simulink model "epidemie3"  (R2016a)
settings: Solver=FixedStepDiscrete  StartTime=0.0  StopTime=300  FixedStep=1  RelTol=1e-3
InitFcn:
  | init_epidemie
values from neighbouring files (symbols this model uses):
  dt = block.DialogPrm(4).Data    [sfun_oven.m]
  m = 1.0    (= 1)    [init_pendelStange.m]
undefined symbols (not defined in the file or in its folder): N0, v

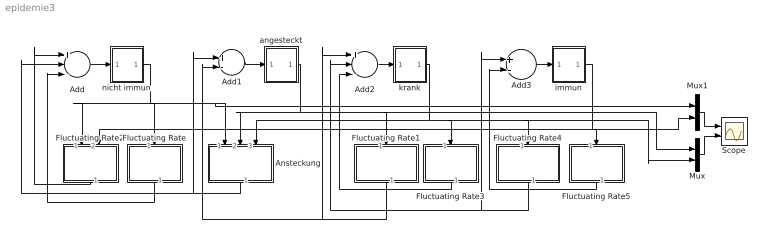
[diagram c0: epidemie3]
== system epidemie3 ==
  Add : Sum  Inputs=+--
  Add1 : Sum  Inputs=+-
  Add2 : Sum  Inputs=+--
  Add3 : Sum  Inputs=+-
  Ansteckung : Subsystem
  Fluctuating Rate : Subsystem
  Fluctuating Rate1 : Subsystem
  Fluctuating Rate2 : Subsystem
  Fluctuating Rate3 : Subsystem
  Fluctuating Rate4 : Subsystem
  Fluctuating Rate5 : Subsystem
  Mux : Mux  Inputs=2
  Mux1 : Mux  Inputs=2
  Scope : Scope  NumInputPorts=2
  angesteckt : Subsystem
  immun : Subsystem
  krank : Subsystem
  nicht immun : Subsystem
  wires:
  Add/1 -> nicht immun/1(In)
  nicht immun/1(Out) -> Ansteckung/1(N), Mux1/1, Fluctuating Rate/1(N), Fluctuating Rate2/1(N)
  immun/1(Out) -> Mux1/2, Fluctuating Rate5/1(N), Fluctuating Rate2/2(I)
  Fluctuating Rate2/1(dn) -> Add/1
  angesteckt/1(Out) -> Ansteckung/2(A), Mux/1, Fluctuating Rate1/1(N)
  krank/1(Out) -> Ansteckung/3(K), Mux/2, Fluctuating Rate4/1(N), Fluctuating Rate3/1(N)
  Ansteckung/1(a) -> Add/2, Add1/1
  Add1/1 -> angesteckt/1(In)
  Fluctuating Rate1/1(dn) -> Add2/1, Add1/2
  Add2/1 -> krank/1(In)
  Fluctuating Rate4/1(dn) -> Add3/1, Add2/2
  Fluctuating Rate3/1(dn) -> Add2/3
  Mux1/1 -> Scope/1
  Mux/1 -> Scope/2
  Add3/1 -> immun/1(In)
  Fluctuating Rate/1(dn) -> Add/3
  Fluctuating Rate5/1(dn) -> Add3/2

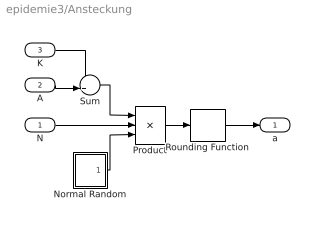
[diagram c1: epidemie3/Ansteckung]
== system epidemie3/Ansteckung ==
  N : Inport
  A : Inport  Port=2
  K : Inport  Port=3
  Normal Random : Subsystem
  Product : Product  Inputs=3
  Rounding Function : Rounding  Operator=round
  Sum : Sum  Inputs=++|
  a : Outport
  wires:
  Sum/1 -> Product/1
  Product/1 -> Rounding Function/1
  K/1 -> Sum/1
  A/1 -> Sum/2
  N/1 -> Product/2
  Normal Random/1(Out1) -> Product/3
  Rounding Function/1 -> a/1

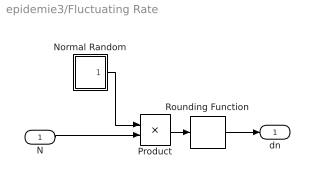
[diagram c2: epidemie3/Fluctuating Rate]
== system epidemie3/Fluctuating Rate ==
  N : Inport
  Normal Random : Subsystem
  Product : Product
  Rounding Function : Rounding  Operator=round
  dn : Outport
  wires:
  Product/1 -> Rounding Function/1
  Normal Random/1(Out1) -> Product/1
  N/1 -> Product/2
  Rounding Function/1 -> dn/1

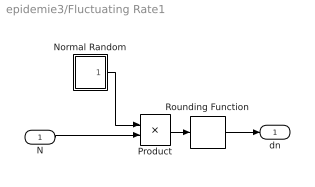
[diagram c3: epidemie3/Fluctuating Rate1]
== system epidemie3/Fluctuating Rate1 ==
  N : Inport
  Normal Random : Subsystem
  Product : Product
  Rounding Function : Rounding  Operator=round
  dn : Outport
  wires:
  Rounding Function/1 -> dn/1
  N/1 -> Product/2
  Normal Random/1(Out1) -> Product/1
  Product/1 -> Rounding Function/1

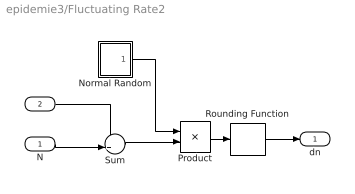
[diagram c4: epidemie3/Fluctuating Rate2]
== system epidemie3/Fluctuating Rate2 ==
  N : Inport
  I : Inport  Port=2
  Normal Random : Subsystem
  Product : Product
  Rounding Function : Rounding  Operator=round
  Sum : Sum  Inputs=++|
  dn : Outport
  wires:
  Rounding Function/1 -> dn/1
  Normal Random/1(Out1) -> Product/1
  Product/1 -> Rounding Function/1
  N/1 -> Sum/2
  Sum/1 -> Product/2
  I/1 -> Sum/1

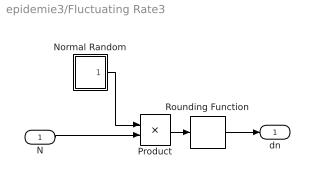
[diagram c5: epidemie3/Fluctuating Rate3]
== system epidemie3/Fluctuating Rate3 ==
  N : Inport
  Normal Random : Subsystem
  Product : Product
  Rounding Function : Rounding  Operator=round
  dn : Outport
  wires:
  Rounding Function/1 -> dn/1
  N/1 -> Product/2
  Normal Random/1(Out1) -> Product/1
  Product/1 -> Rounding Function/1

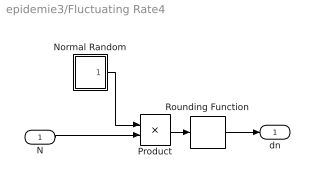
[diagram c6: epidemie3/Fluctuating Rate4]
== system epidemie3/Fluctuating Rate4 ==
  N : Inport
  Normal Random : Subsystem
  Product : Product
  Rounding Function : Rounding  Operator=round
  dn : Outport
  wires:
  Product/1 -> Rounding Function/1
  Normal Random/1(Out1) -> Product/1
  N/1 -> Product/2
  Rounding Function/1 -> dn/1

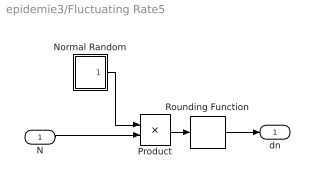
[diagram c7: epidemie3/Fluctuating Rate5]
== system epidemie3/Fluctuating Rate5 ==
  N : Inport
  Normal Random : Subsystem
  Product : Product
  Rounding Function : Rounding  Operator=round
  dn : Outport
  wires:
  Rounding Function/1 -> dn/1
  N/1 -> Product/2
  Normal Random/1(Out1) -> Product/1
  Product/1 -> Rounding Function/1

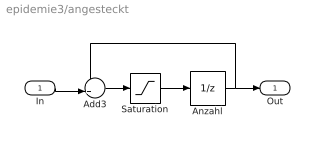
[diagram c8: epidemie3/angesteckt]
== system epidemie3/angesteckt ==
  In : Inport
  Add3 : Sum  Inputs=++|
  Anzahl : UnitDelay  InitialCondition=N0  SampleTime=-1
  Saturation : Saturate  UpperLimit=Inf  LowerLimit=0
  Out : Outport
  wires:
  In/1 -> Add3/2
  Anzahl/1 -> Out/1, Add3/1
  Add3/1 -> Saturation/1
  Saturation/1 -> Anzahl/1

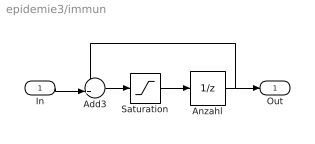
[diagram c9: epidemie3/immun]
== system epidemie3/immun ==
  In : Inport
  Add3 : Sum  Inputs=++|
  Anzahl : UnitDelay  InitialCondition=N0  SampleTime=-1
  Saturation : Saturate  UpperLimit=Inf  LowerLimit=0
  Out : Outport
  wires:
  Saturation/1 -> Anzahl/1
  Add3/1 -> Saturation/1
  Anzahl/1 -> Add3/1, Out/1
  In/1 -> Add3/2

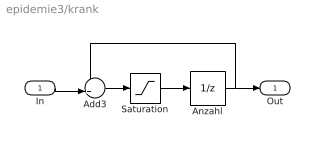
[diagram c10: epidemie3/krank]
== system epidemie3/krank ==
  In : Inport
  Add3 : Sum  Inputs=++|
  Anzahl : UnitDelay  InitialCondition=N0  SampleTime=-1
  Saturation : Saturate  UpperLimit=Inf  LowerLimit=0
  Out : Outport
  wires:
  In/1 -> Add3/2
  Anzahl/1 -> Out/1, Add3/1
  Add3/1 -> Saturation/1
  Saturation/1 -> Anzahl/1

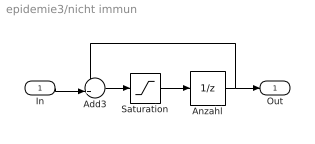
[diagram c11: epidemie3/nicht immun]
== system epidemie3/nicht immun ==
  In : Inport
  Add3 : Sum  Inputs=++|
  Anzahl : UnitDelay  InitialCondition=N0  SampleTime=-1
  Saturation : Saturate  UpperLimit=Inf  LowerLimit=0
  Out : Outport
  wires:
  Saturation/1 -> Anzahl/1
  Add3/1 -> Saturation/1
  Anzahl/1 -> Add3/1, Out/1
  In/1 -> Add3/2

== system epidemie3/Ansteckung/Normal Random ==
  Bias : Bias  Bias=m
  Constant : Constant
  Gain : Gain  Gain=sqrt(v)
  randn : MATLABFcn  MATLABFcn=randn  SampleTime=dt
  Out1 : Outport
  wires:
  Bias/1 -> Out1/1
  Gain/1 -> Bias/1
  randn/1 -> Gain/1
  Constant/1 -> randn/1

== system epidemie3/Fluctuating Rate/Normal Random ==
  Bias : Bias  Bias=m
  Constant : Constant
  Gain : Gain  Gain=sqrt(v)
  randn : MATLABFcn  MATLABFcn=randn  SampleTime=dt
  Out1 : Outport
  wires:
  Bias/1 -> Out1/1
  Gain/1 -> Bias/1
  randn/1 -> Gain/1
  Constant/1 -> randn/1

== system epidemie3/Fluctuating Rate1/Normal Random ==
  Bias : Bias  Bias=m
  Constant : Constant
  Gain : Gain  Gain=sqrt(v)
  randn : MATLABFcn  MATLABFcn=randn  SampleTime=dt
  Out1 : Outport
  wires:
  Constant/1 -> randn/1
  randn/1 -> Gain/1
  Gain/1 -> Bias/1
  Bias/1 -> Out1/1

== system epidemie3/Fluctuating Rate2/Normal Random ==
  Bias : Bias  Bias=m
  Constant : Constant
  Gain : Gain  Gain=sqrt(v)
  randn : MATLABFcn  MATLABFcn=randn  SampleTime=dt
  Out1 : Outport
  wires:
  Constant/1 -> randn/1
  randn/1 -> Gain/1
  Gain/1 -> Bias/1
  Bias/1 -> Out1/1

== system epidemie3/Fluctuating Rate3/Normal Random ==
  Bias : Bias  Bias=m
  Constant : Constant
  Gain : Gain  Gain=sqrt(v)
  randn : MATLABFcn  MATLABFcn=randn  SampleTime=dt
  Out1 : Outport
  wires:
  Constant/1 -> randn/1
  randn/1 -> Gain/1
  Gain/1 -> Bias/1
  Bias/1 -> Out1/1

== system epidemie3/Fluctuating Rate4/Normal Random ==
  Bias : Bias  Bias=m
  Constant : Constant
  Gain : Gain  Gain=sqrt(v)
  randn : MATLABFcn  MATLABFcn=randn  SampleTime=dt
  Out1 : Outport
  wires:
  Bias/1 -> Out1/1
  Gain/1 -> Bias/1
  randn/1 -> Gain/1
  Constant/1 -> randn/1

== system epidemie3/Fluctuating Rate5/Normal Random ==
  Bias : Bias  Bias=m
  Constant : Constant
  Gain : Gain  Gain=sqrt(v)
  randn : MATLABFcn  MATLABFcn=randn  SampleTime=dt
  Out1 : Outport
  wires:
  Constant/1 -> randn/1
  randn/1 -> Gain/1
  Gain/1 -> Bias/1
  Bias/1 -> Out1/1
